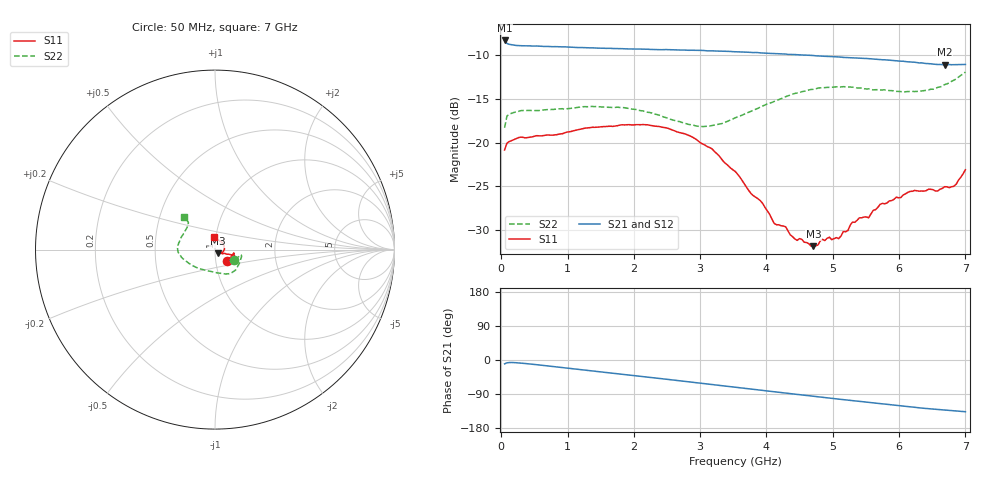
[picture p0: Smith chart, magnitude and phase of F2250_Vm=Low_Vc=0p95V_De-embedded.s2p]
! Integrated Device Technology
! Corporate Headquarters
! 6024 Silver Creek Valley Road
! San Jose, CA 95138  USA
! Phone:  1-408-284-8200
! Toll Free:  1-800-223-1366
! Webpage:  http://www.idt.com/
! Timing and RF Division
! 515 Groton Road, Suite 102
! Westford, MA 01886-6024
! Device:  F2250
! Description: Voltage Variable RF Attenuator
! Frequency:  50.0 -  6000.00 MHz
! Package:  3x3 mm Thin QFN Plastic Package: 16 pin
! Ports:  2 RF, 3 DC
!  Pin  1  = GND
!  Pin  2  = NC
!  Pin  3  = RF1  = Port 1
!  Pin  4  = NC
!  Pin  5  = GND
!  Pin  6  = GND
!  Pin  7  = GND
!  Pin  8  = GND
!  Pin  9  = NC
!  Pin 10  = RF2  = Port 2
!  Pin 11  = NC
!  Pin 12  = GND
!  Pin 13  = GND
!  Pin 14  = VCNTRL
!  Pin 15  = VDD
!  Pin 16  = VMODE
! Vcntrl:  0.950 Volts
! Vmode:  +0.000 Volts
! Vdd:  +3.30  Volts
! Current:  1.183 mA
! Data:  The device was measured on a the F2250 evaluation board which has
!  individual transmission lines to the RF pins.  Data was collected
!  using a calibrated network analyzer.  The evaluation board was
!  de-embedded using a TRL calibration technique.
!  The reference plane is the edge of the package pin.
! Misc:  SN 10
!  Action Tracker AT0258
! Date Measured:  2014-11-26
! Date:  2015-10-15  MJV
! Note:
!  Integrated Device Technology supplies this data as a sample of measured
!  data at the package pin for this product.  Your particular data for this
!  product may vary.
!  Data was taken at 25 degrees C.
!  Integrated Device Technology reserves the right to change this data at anytime.
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# GHz S dB R 50
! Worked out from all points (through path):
!   201 points, 50 MHz to 7 GHz, reference 50 ohm
!   highest |S21| = -8.29 dB at 50 MHz (marker M1); lowest = -11.1 dB at 6.687 GHz (marker M2)
!   group delay of S21, straight-line fit = 54.5 ps
!   lowest |S11| = -31.9 dB at 4.707 GHz (marker M3), VSWR 1.05, Z = 51.4 - j2.19 ohm
!   |S11| at or under -10 dB: start of sweep to end of sweep
!   |S22| runs from -18.3 to -11.9 dB; largest |S21 - S12| = 0.0011
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0.05  -20.83 -44.8  -8.29 -10.2  -8.28 -10.2  -18.29 -27.0
0.08475  -20.06 -23.1  -8.63 -7.5  -8.63 -7.5  -16.96 -14.8
0.189  -19.65 -12.4  -8.82 -6.8  -8.83 -6.8  -16.54 -11.5
1.2315  -18.38 -21.5  -9.10 -26.1  -9.09 -26.1  -15.88 -42.0
2.37825  -18.14 -20.1  -9.34 -48.5  -9.34 -48.5  -16.83 -69.9
3.0385  -20.16 -18.3  -9.43 -61.9  -9.44 -61.9  -18.15 -101.6
3.525  -23.27 -21.3  -9.58 -71.8  -9.59 -71.8  -17.16 -130.9
3.942  -26.96 -29.4  -9.73 -80.3  -9.73 -80.3  -15.80 -150.8
4.11575  -29.24 -36.0  -9.78 -83.8  -9.78 -83.8  -15.27 -157.7
4.2895  -29.64 -43.4  -9.84 -87.3  -9.85 -87.3  -14.72 -163.2
4.46325  -31.19 -51.0  -9.92 -90.8  -9.92 -90.8  -14.31 -168.0
4.7065  -31.85 -56.4  -10.01 -95.7  -10.02 -95.7  -13.89 -173.9
4.94975  -30.83 -53.0  -10.11 -100.5  -10.11 -100.5  -13.65 -179.2
5.08875  -30.99 -49.1  -10.17 -103.2  -10.17 -103.3  -13.62 177.6
5.29725  -29.09 -39.4  -10.28 -107.2  -10.29 -107.2  -13.64 173.0
5.5405  -28.61 -28.5  -10.37 -112.0  -10.38 -112.0  -13.83 166.7
5.71425  -27.06 -22.1  -10.48 -115.3  -10.47 -115.3  -13.96 162.1
5.85325  -26.67 -15.2  -10.54 -117.9  -10.55 -118.0  -14.03 158.5
6.166  -25.58 2.4  -10.74 -123.7  -10.73 -123.8  -14.13 148.4
6.68725  -25.04 50.7  -11.07 -131.9  -11.06 -132.0  -13.34 134.1
6.82625  -25.00 67.4  -11.06 -133.8  -11.06 -133.9  -12.84 133.9
7  -23.09 93.3  -11.04 -136.5  -11.03 -136.6  -11.91 133.7
